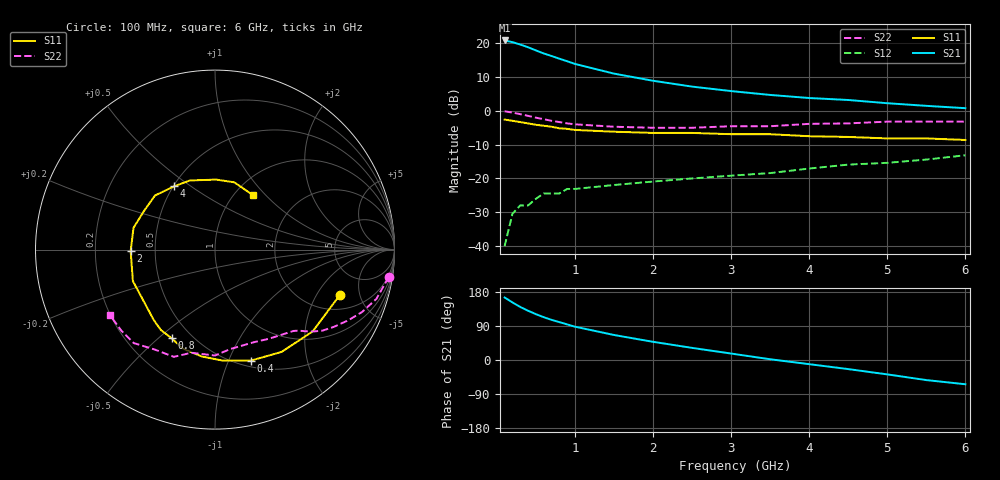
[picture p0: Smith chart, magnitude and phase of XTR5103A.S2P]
! HXTR-5103  (2N6741) Common Emitter
! Vce=18V  Ic=30mA
# ghz s ma r 50
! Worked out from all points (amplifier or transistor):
!   20 points, 100 MHz to 6 GHz, reference 50 ohm
!   highest |S21| = 20.7 dB at 100 MHz (marker M1)
!   |S21| within 3 dB of that: start of sweep to 506.7 MHz
!   unconditionally stable (mu >= 1): 1.976 GHz to 3.939 GHz
!   at 400 MHz: K = 0.28, MSG = 23.3 dB, |S12| = -28.0 dB
!   at 1.5 GHz: K = 0.86, MSG = 16.4 dB, |S12| = -21.9 dB
!   at 6 GHz: K = 0.81, MSG = 7.0 dB, |S12| = -13.2 dB
!   S11 on the Smith chart (normalised r, x): 100 MHz: 2.88, -3.23; 400 MHz: 0.57, -1.21; 800 MHz: 0.39, -0.55; 2 GHz: 0.36, -0.01; 4 GHz: 0.50, +0.43; 6 GHz: 1.21, +0.85
0.1  0.74 -20.0  10.9 165.0  0.01 79.0  0.98 -9.0
0.2  0.71 -40.0  10.3 152.0  0.03 68.0  0.94 -17.0
0.3  0.68 -57.0  9.49 140.0  0.04 62.0  0.89 -23.0
0.4  0.65 -72.0  8.65 130.0  0.04 55.0  0.84 -28.0
0.5  0.62 -86.0  7.77 121.0  0.05 49.0  0.79 -33.0
0.6  0.6 -97.0  7.01 113.0  0.06 44.0  0.75 -37.0
0.7  0.58 -108.0  6.43 106.0  0.06 41.0  0.71 -40.0
0.8  0.55 -116.0  5.87 100.0  0.06 38.0  0.68 -42.0
0.9  0.54 -124.0  5.38 94.0  0.07 35.0  0.65 -44.0
1  0.52 -131.0  4.91 88.0  0.07 33.0  0.63 -46.0
1.5  0.49 -159.0  3.53 66.0  0.08 25.0  0.58 -59.0
2  0.47 -179.0  2.77 48.0  0.09 22.0  0.56 -67.0
2.5  0.47 165.0  2.27 32.0  0.1 18.0  0.56 -81.0
3  0.45 151.0  1.95 17.0  0.11 15.0  0.59 -90.0
3.5  0.45 138.0  1.71 2.0  0.12 10.0  0.59 -103.0
4  0.42 123.0  1.54 -11.0  0.14 4.0  0.64 -111.0
4.5  0.41 110.0  1.44 -24.0  0.16 1.0  0.65 -121.0
5  0.39 89.0  1.29 -38.0  0.17 -6.0  0.69 -131.0
5.5  0.39 74.0  1.18 -53.0  0.19 -12.0  0.69 -139.0
6  0.37 55.0  1.09 -64.0  0.22 -17.0  0.69 -148.0
